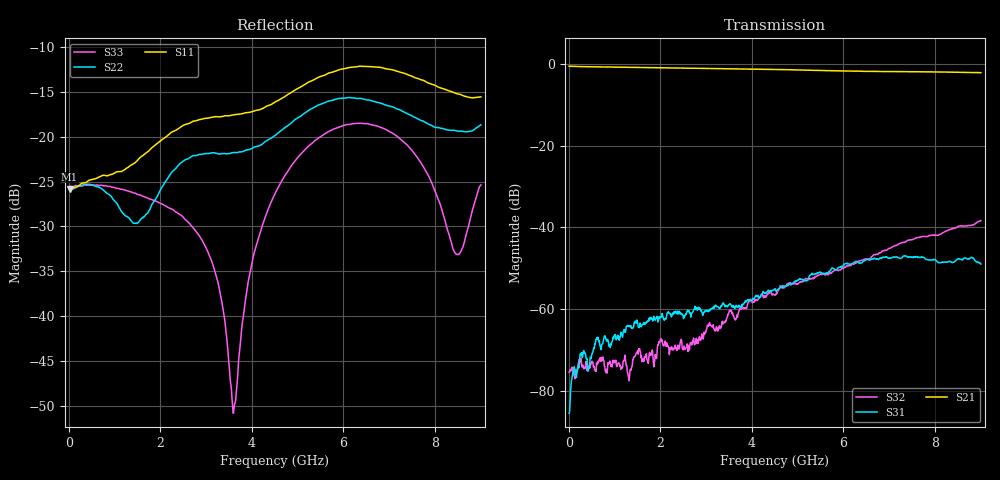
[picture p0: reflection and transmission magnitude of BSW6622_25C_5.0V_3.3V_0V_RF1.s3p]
!Agilent Technologies,N5230C,MY49001333,A.09.33.09
!Agilent N5230C: A.09.33.09
!Date: Monday, September 23, 2024 11:08:53
!Correction: S11(Full 3 Port(1,2,3))
!S12(Full 3 Port(1,2,3))
!S13(Full 3 Port(1,2,3))
!S21(Full 3 Port(1,2,3))
!S22(Full 3 Port(1,2,3))
!S23(Full 3 Port(1,2,3))
!S31(Full 3 Port(1,2,3))
!S32(Full 3 Port(1,2,3))
!S33(Full 3 Port(1,2,3))
!S3P File: Measurements: <S11,S12,S13>,
!<S21,S22,S23>,
!<S31,S32,S33>:
# Hz S  MA  R 50
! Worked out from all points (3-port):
!   901 points, 10 MHz to 9.01 GHz, reference 50 ohm
!   strongest paths, dB at 10 MHz, 2.26 GHz, 4.51 GHz, 6.76 GHz, 9.01 GHz:
!     S21: -0.6, -1.0, -1.4, -1.9, -2.2
!     S31: -85.5, -61.4, -55.0, -47.8, -49.0
!     S32: -75.4, -70.0, -56.6, -46.6, -38.4
!   lowest |S11| = -25.8 dB at 20 MHz (marker M1), VSWR 1.11, Z = 55.4 - j0.186 ohm
!   |S11| at or under -10 dB: start of sweep to end of sweep
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1e7  0.05128 -1.5  0.9331 -2.4  9.842e-05 28.2
     0.9341 -2.4  0.05164 -0.3  0.0001442 -37.8
     5.325e-05 83.2  0.0001689 -81.3  0.05139 -5.2
2e7  0.05127 -1.9  0.9328 -3.0  0.000113 4.5
     0.9335 -3.0  0.05159 -0.7  0.0001927 -22.2
     5.557e-05 58.0  0.0001699 -77.6  0.05212 -4.8
1.63e9  0.0788 153.9  0.8971 -170.5  0.0005493 -72.8
        0.8971 -170.5  0.03543 149.7  0.0002141 19.4
        0.0006549 -62.4  0.0002484 -14.6  0.04655 -150.2
2.53e9  0.1167 36.5  0.8848 95.9  0.0008797 -159.9
        0.8838 95.9  0.07394 13.5  0.0003477 -65.5
        0.0007989 -166.7  0.0003257 -85.5  0.03495 124.1
3.37e9  0.1303 -59.5  0.8729 8.5  0.001058 127.1
        0.8709 8.6  0.08078 -72.1  0.0007657 -113.7
        0.001172 134.8  0.0006599 -126.1  0.01119 45.7
4.51e9  0.1564 171.6  0.8558 -110.1  0.001658 35.1
        0.852 -110.0  0.1017 171.0  0.001756 118.7
        0.00178 35.7  0.001472 118.0  0.04813 156.4
5.92e9  0.2373 23.4  0.8223 103.3  0.003311 -104.1
        0.818 103.6  0.1639 10.0  0.002953 -26.6
        0.003255 -103.6  0.003012 -27.4  0.1136 57.0
6.94e9  0.2397 -74.9  0.8073 -2.6  0.004198 136.6
        0.8039 -2.3  0.1502 -104.5  0.005106 -127.2
        0.004345 134.5  0.005233 -128.7  0.1097 -11.5
7.87e9  0.1995 -165.5  0.7958 -100.4  0.004093 28.3
        0.7958 -100.0  0.1177 142.3  0.007459 131.0
        0.003977 27.5  0.007884 130.9  0.06032 -66.8
9.01e9  0.1672 69.1  0.7777 139.7  0.003508 -106.5
        0.7782 140.0  0.1167 4.1  0.01124 20.8
        0.003564 -115.6  0.01206 20.3  0.05399 -16.9
